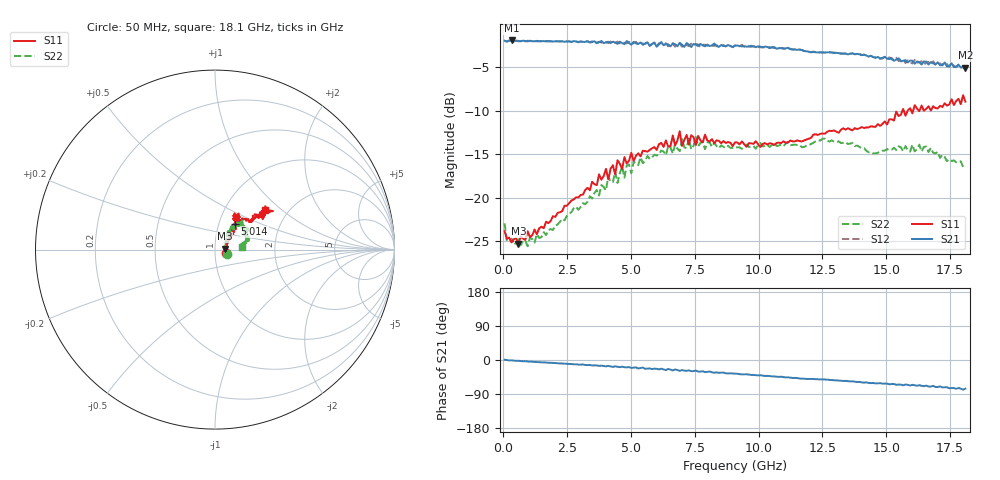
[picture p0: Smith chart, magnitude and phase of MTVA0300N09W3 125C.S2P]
! Network Analyzer HP8720D.06.14 Serial No. US36140669
!  7 Jul 2005  13:00:25
! Frequency  S11  S21  S12  S22
# HZ  S  DB R 50
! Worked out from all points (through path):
!   201 points, 50 MHz to 18.1 GHz, reference 50 ohm
!   highest |S21| = -1.92 dB at 320.8 MHz (marker M1); lowest = -5.1 dB at 18.1 GHz (marker M2)
!   group delay of S21, straight-line fit = 11.7 ps
!   lowest |S11| = -25.3 dB at 591.5 MHz (marker M3), VSWR 1.12, Z = 55.7 + j0.519 ohm
!   |S11| at or under -10 dB: start of sweep to 15.63 GHz; 15.69 GHz to 15.84 GHz (149.6 MHz wide, 0.949 % of centre); 15.97805 GHz to 16.053 GHz (74.94 MHz wide, 0.468 % of centre)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
!   |S22| runs from -25.6 to -13.0 dB; largest |S21 - S12| = 0.044
!   S11 on the Smith chart (normalised r, x): 50 MHz: 1.13, -0.05; 5.014 GHz: 1.20, +0.35; 18.1 GHz: 1.54, +0.78
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5e7  -23.84 -19.7  -1.95 0.7  -1.99 0.7  -22.94 -20.0
1.4025e8  -24.72 -10.5  -2.06 -0.2  -2.05 -0.3  -24.96 -9.1
3.2075e8  -25.12 -0.2  -1.92 -0.8  -1.97 -0.8  -24.66 -1.4
5.915e8  -25.26 4.9  -1.97 -1.9  -2.03 -2.2  -24.78 7.1
1.22325e9  -23.64 18.0  -2.02 -5.1  -1.98 -4.9  -25.15 15.0
3.1185e9  -19.64 39.8  -2.08 -11.8  -2.12 -12.2  -20.61 45.7
4.021e9  -16.68 46.2  -2.15 -16.8  -2.11 -15.7  -19.15 48.2
4.11125e9  -17.89 47.0  -2.08 -15.5  -2.22 -16.8  -17.49 49.0
4.47225e9  -15.69 44.5  -2.33 -17.8  -2.06 -17.3  -18.29 54.8
4.65275e9  -16.67 45.3  -2.22 -17.6  -2.14 -19.4  -16.33 54.7
5.01375e9  -14.84 51.8  -2.42 -21.0  -2.34 -19.4  -17.18 49.0
6.09675e9  -13.84 52.4  -2.37 -24.8  -2.25 -24.6  -15.03 48.7
6.7285e9  -13.98 59.8  -2.35 -24.8  -2.64 -25.4  -13.87 44.6
6.909e9  -12.36 56.9  -2.20 -28.5  -2.23 -26.6  -14.64 45.1
6.99925e9  -14.04 56.7  -2.41 -26.6  -2.64 -28.6  -13.26 45.7
7.36025e9  -12.80 52.3  -2.69 -29.5  -2.30 -28.9  -14.42 48.6
7.54075e9  -13.94 55.2  -2.42 -27.9  -2.34 -31.1  -13.00 47.0
9.075e9  -13.63 57.7  -2.53 -36.0  -2.49 -36.3  -14.17 35.4
1.21435e10  -12.75 48.1  -3.25 -50.1  -3.20 -50.4  -13.68 34.7
1.512175e10  -10.98 38.2  -4.05 -64.1  -3.86 -63.8  -14.53 25.0
1.6295e10  -10.04 32.6  -4.41 -66.4  -4.41 -69.8  -13.89 19.6
1.81e10  -8.96 38.4  -5.06 -75.7  -5.24 -76.6  -16.27 6.2
